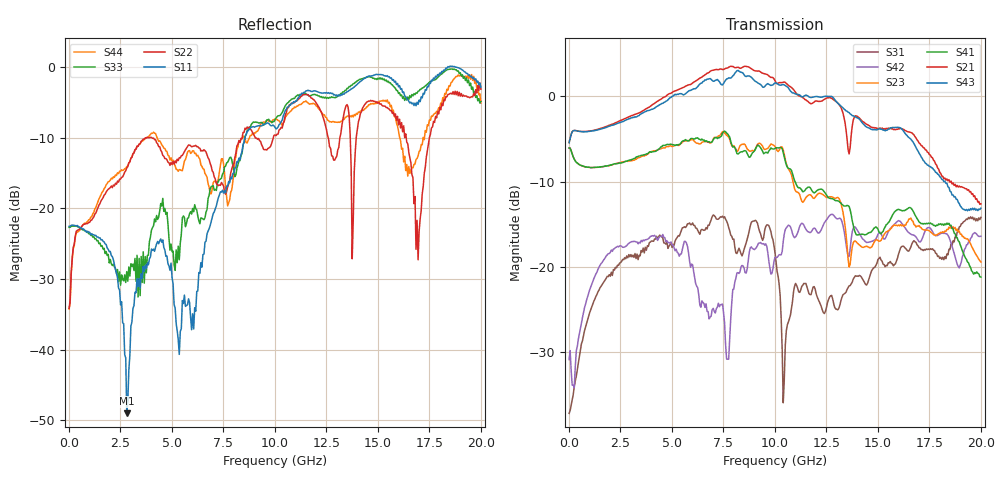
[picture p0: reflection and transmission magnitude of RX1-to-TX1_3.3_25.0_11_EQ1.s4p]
!Agilent Technologies,N5225A,MY51451112,A.09.50.13
!Agilent N5225A: A.09.50.13
!Date: Wednesday, January 31, 2018 11:02:44
!Correction: S11(Full 4 Port(1,2,3,4))
!S12(Full 4 Port(1,2,3,4))
!S13(Full 4 Port(1,2,3,4))
!S14(Full 4 Port(1,2,3,4))
!S21(Full 4 Port(1,2,3,4))
!S22(Full 4 Port(1,2,3,4))
!S23(Full 4 Port(1,2,3,4))
!S24(Full 4 Port(1,2,3,4))
!S31(Full 4 Port(1,2,3,4))
!S32(Full 4 Port(1,2,3,4))
!S33(Full 4 Port(1,2,3,4))
!S34(Full 4 Port(1,2,3,4))
!S41(Full 4 Port(1,2,3,4))
!S42(Full 4 Port(1,2,3,4))
!S43(Full 4 Port(1,2,3,4))
!S44(Full 4 Port(1,2,3,4))
!S4P File: Measurements: <S11,S12,S13,S14>,
!<S21,S22,S23,S24>,
!<S31,S32,S33,S34>,
!<S41,S42,S43,S44>:
# Hz S  RI  R 50
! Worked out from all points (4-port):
!   401 points, 10 MHz to 20 GHz, reference 50 ohm
!   strongest paths, dB at 10 MHz, 5.008 GHz, 10.01 GHz, 15 GHz, 20 GHz:
!     S43: -5.4, 0.0, 1.6, -3.9, -13.1
!     S21: -5.4, 0.4, 1.8, -3.8, -12.6
!     S41: -6.1, -5.7, -6.1, -15.6, -21.2
!     S23: -6.1, -5.9, -5.9, -16.9, -19.4
!     S42: -30.8, -17.4, -18.9, -16.2, -16.4
!     S31: -37.1, -17.7, -18.3, -19.1, -14.2
!   lowest |S11| = -49.0 dB at 2.809 GHz (marker M1), VSWR 1.01, Z = 49.7 - j0.215 ohm
!   |S11| at or under -10 dB: start of sweep to 8.544 GHz
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1e7  -0.0745 -0.00305  0.00026 0.000275  0.0138 0.000948  -0.000344 0.000538
     0.5359 0.00657  -0.0136 0.0141  -0.4979 0.00462  0.0263 0.012
     0.0139 0.000767  -0.000113 0.000509  -0.0732 -0.00436  -7.73e-05 0.00041
     -0.4978 0.00507  0.0262 0.0118  0.534 0.00615  -0.0131 0.0143
2.8086e9  -0.00281 -0.00216  0.0166 0.00253  0.0553 0.1036  0.018 0.00015
          0.4532 -0.5937  0.1933 0.00292  -0.1426 0.3912  0.0995 0.0918
          0.056 0.1017  0.0198 0.00312  0.0202 0.0294  0.0215 0.000293
          -0.0881 0.4075  0.0942 0.0947  0.3076 -0.6607  0.1909 -0.0509
5.757125e9  0.0142 0.0151  0.0189 -0.0207  0.118 0.1281  0.0118 -0.0415
            -0.754 -0.8773  0.1244 -0.244  0.4981 0.2322  0.1216 -0.017
            0.1066 0.1438  0.029 -0.0279  0.0703 0.048  0.0169 -0.052
            0.5445 0.0617  0.1311 -0.0171  -0.9455 -0.4681  0.0448 -0.2452
8.355825e9  -0.0328 0.2376  -0.00421 -0.0282  0.1229 0.0552  -0.0113 -0.017
            -1.004 1.058  -0.0759 0.3028  0.2582 -0.4505  -0.0373 0.0804
            0.1036 0.0598  -0.00542 -0.0152  0.0051 0.2366  0.00279 -0.0183
            0.00416 -0.4727  -0.0172 0.0989  -0.2786 1.35  0.2042 0.2358
1.050475e10  0.1221 0.4776  -0.0281 -0.0332  0.0426 0.0174  -0.0489 -0.00357
             0.7447 0.9452  0.3174 0.3326  -0.3689 -0.2115  0.0543 0.1725
             0.0226 0.0267  -0.0366 -0.0299  0.1789 0.5024  -0.0534 -0.00813
             -0.4156 -0.0119  0.0731 0.1485  1.104 0.3329  0.4294 -0.0962
1.28036e10  0.291 0.5835  -0.0379 -0.00229  0.0313 0.0516  -0.0315 0.013
            0.8797 -0.3861  0.1855 0.1431  -0.2486 0.0629  0.1972 0.1014
            0.0351 0.055  -0.03 -0.00685  0.4239 0.4385  -0.0439 0.00451
            -0.1559 0.1967  0.1794 0.0958  0.3253 -0.9317  0.2064 -0.356
2e10  0.7165 0.0565  0.0229 0.0348  -0.0811 0.1721  0.0343 0.0208
      -0.0789 0.2208  0.6926 0.0774  0.1067 0.00867  0.1493 0.0442
      -0.0849 0.1758  0.00638 0.0477  0.5705 -0.0329  0.0479 0.0207
      0.038 -0.0786  0.1444 0.0454  0.1639 0.1486  -0.1529 -0.5353
